FUNCTION_BLOCK MIS_ProfileVelocity
VAR_INPUT
	eCmd : eCommand;
	rVelocityRpm : REAL; //
	rAccellRpms : REAL; 
END_VAR
VAR_IN_OUT
	stMisMotorLocal : stMisMotor;	
END_VAR
VAR_OUTPUT
	diError : DINT;
	eStat: ESTATUS;
END_VAR
VAR
	TonTimeout: Ton;
END_VAR

IF eCmd = eCommand.Reset THEN
	diError := 0;
	eStat := eStatus.Done;
	RETURN;
END_IF;


CASE eCmd OF
	eCommand.Run:
		stMisMotorLocal.udiTargetAccel := any_to_udint(rAccellRpms);
		stMisMotorLocal.diTargetVel := ANY_TO_DINT(rVelocityRpm * ANY_TO_REAL(stMisMotorLocal.diRpmConversion));
END_CASE;

END_FUNCTION_BLOCK
